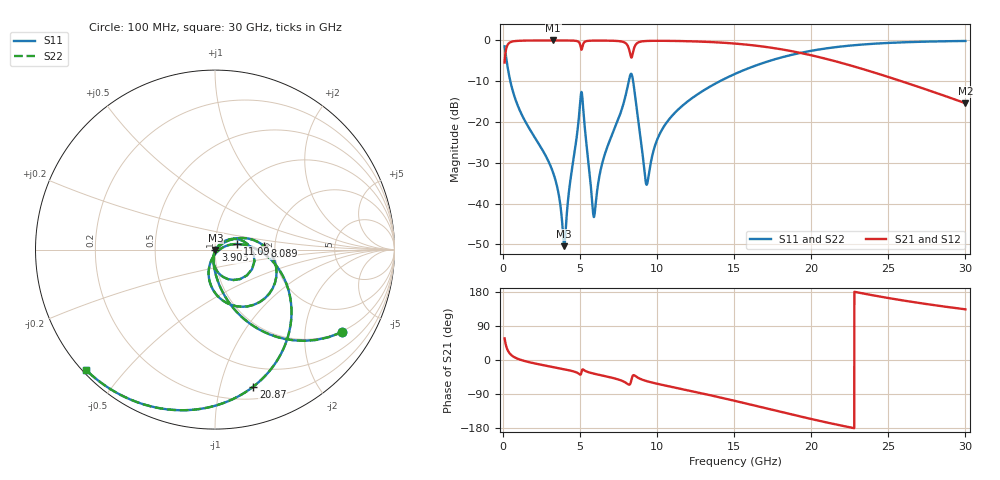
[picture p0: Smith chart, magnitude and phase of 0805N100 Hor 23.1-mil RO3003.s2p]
# GHz S MA R 50
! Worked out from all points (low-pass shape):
!   3201 points, 100 MHz to 30 GHz, reference 50 ohm
!   highest |S21| = -0.02 dB at 3.249 GHz (marker M1); lowest = -15.4 dB at 30 GHz (marker M2)
!   |S21| within 3 dB of the highest: 157.5 MHz to 8.229 GHz (8.072 GHz wide, 192 % of centre); 8.427 GHz to 19.23 GHz (10.8 GHz wide, 78.1 % of centre)
!   lowest |S11| = -50.4 dB at 3.968 GHz (marker M3), VSWR 1.01, Z = 50.3 - j0.153 ohm
!   |S11| at or under -10 dB: 470.1 MHz to 8.153 GHz (7.683 GHz wide, 178 % of centre); 8.439 GHz to 14.07 GHz (5.632 GHz wide, 50 % of centre)
!   |S22| runs from -50.4 to -0.1 dB; largest |S21 - S12| = 0
!   S11 on the Smith chart (normalised r, x): 100 MHz: 0.97, -3.10; 3.903 GHz: 1.00, -0.01; 8.089 GHz: 1.76, +0.07; 11.09 GHz: 1.28, +0.08; 20.87 GHz: 0.31, -1.27; 30 GHz: 0.01, -0.40
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0.1  0.8445 -33.0  0.5351 57.0  0.5351 57.0  0.8445 -33.0
0.3522812  0.4074 -68.1  0.9126 21.8  0.9126 21.8  0.4074 -68.1
0.660625  0.2293 -80.6  0.9725 9.1  0.9725 9.1  0.2293 -80.6
3.248844  0.02389 -103.6  0.9974 -18.8  0.9974 -18.8  0.02389 -103.6
3.61325  0.01286 -100.5  0.9973 -21.6  0.9973 -21.6  0.01286 -100.5
3.902906  0.003985 -68.0  0.997 -23.9  0.997 -23.9  0.003985 -68.0
3.968313  0.003005 -30.4  0.9969 -24.5  0.9969 -24.5  0.003005 -30.4
5.089563  0.2334 -28.0  0.7669 -32.2  0.7669 -32.2  0.2334 -28.0
5.781  0.01045 -77.8  0.9921 -34.9  0.9921 -34.9  0.01045 -77.8
5.911812  0.00693 -21.6  0.9931 -36.2  0.9931 -36.2  0.00693 -21.6
6.491125  0.03414 38.7  0.9933 -41.4  0.9933 -41.4  0.03414 38.7
8.088906  0.2763 3.7  0.8595 -63.4  0.8595 -63.4  0.2763 3.7
8.434625  0.3204 -73.8  0.7162 -40.5  0.7162 -40.5  0.3204 -73.8
8.668219  0.1494 -103.6  0.9145 -44.6  0.9145 -44.6  0.1494 -103.6
9.29425  0.01715 -52.4  0.9826 -55.5  0.9826 -55.5  0.01715 -52.4
10.06978  0.06522 18.3  0.9881 -63.3  0.9881 -63.3  0.06522 18.3
11.08825  0.1261 14.3  0.9841 -72.3  0.9841 -72.3  0.1261 14.3
15.05  0.3882 -19.1  0.9132 -107.9  0.9132 -107.9  0.3882 -19.1
20.03956  0.7476 -66.8  0.654 -156.1  0.654 -156.1  0.7476 -66.8
20.87116  0.7925 -74.4  0.5996 -163.7  0.5996 -163.7  0.7925 -74.4
25.01978  0.9305 -107.2  0.355 163.4  0.355 163.4  0.9305 -107.2
30  0.9829 -136.8  0.1699 133.7  0.1699 133.7  0.9829 -136.8
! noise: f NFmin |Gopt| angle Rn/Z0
0.1  0.0007185  0.9142  0.9888  0.001846
3.417  0.006689  0.7193  21.2  0.004561
6.743  0.01539  0.7608  40.87  0.01148
10.06  0.0226  0.7664  59.45  0.01492
13.39  0.02281  0.7151  75.98  0.009983
16.7  0.02854  0.7278  91.05  0.0105
20.03  0.0368  0.7564  105  0.01169
23.35  0.04862  0.7935  118.1  0.01332
26.67  0.06651  0.8358  130.8  0.01539
30  0.09552  0.879  143.3  0.01758
